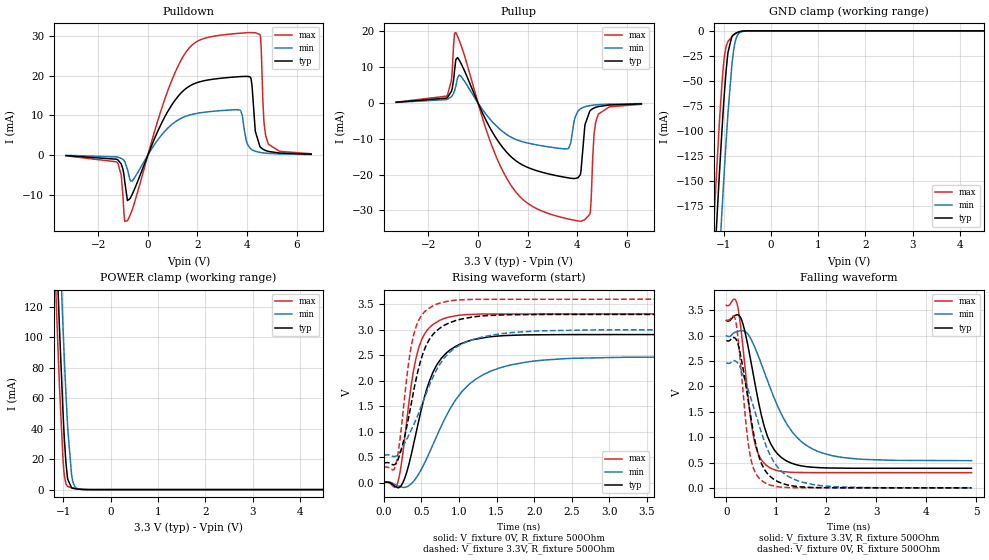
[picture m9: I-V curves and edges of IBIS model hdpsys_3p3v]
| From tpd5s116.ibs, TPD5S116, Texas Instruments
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[Model]   hdpsys_3p3v
Model_type   3-state
Polarity   Non-Inverting
Vmeas = 1.65
Vref = 3.3
Cref = 15pF
Rref = 500
|   typ   min   max
|   (nom PVT)   (slow PVT)   (fast PVT)
C_comp   1.1241p   1.0342p   1.3025p
|C_comp (High state)   1.1241p   1.0342p   1.3025p
|C_comp (Low state)   1.0197p   0.970p   1.0858p
| Where nom  PVT is Nominal Process, 3.3V, 27C
|   Fast PVT is Strong Process,  3.6V, -40C
|   Slow PVT is Weak Process,   3.0V, 125C
[Voltage Range]   3.3   3   3.6
[Temperature Range]   27   125   -40
[Pullup Reference]   3.3   3   3.6
[Pulldown Reference]   -0   -0   -0
[Power Clamp Reference]   3.3   3   3.6
[GND Clamp Reference]   -0   -0   -0
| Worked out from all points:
|   slope of the pulldown table from 0 to 0.495 V, typ, clamps not added: 68 ohm
|   slope of the pullup table from 0 to 0.495 V, typ, clamps not added: 69.7 ohm
|   GND clamp passes 1 mA (typ) near -0.67 V on its own axis
|   POWER clamp passes 1 mA (typ) near -0.81 V on its own axis
|   falling waveform, V_fixture 3.3V, R_fixture 500Ohm: 20-80 % time 394ps typ, 706ps min, 239ps max; typ from 3.3 V to 0.386 V
|   rising waveform, V_fixture 0V, R_fixture 500Ohm: 20-80 % time 342ps typ, 596ps min, 205ps max; typ from 0 V to 2.9 V
|   rising waveform, V_fixture 3.3V, R_fixture 500Ohm: 20-80 % time 285ps typ, 480ps min, 181ps max; typ from 0.386 V to 3.3 V
|   falling waveform, V_fixture 0V, R_fixture 500Ohm: 20-80 % time 325ps typ, 540ps min, 208ps max; typ from 2.91 V to 0 V
[Pulldown]
|   Voltage   I(typ)   I(min)   I(max)
-3.3V     -127.7uA   -60.24uA   -174.8uA
-1.261V   -1.034mA   -454.9uA   -1.695mA
-825mV    -11.44mA   -3.562mA   -16.52mA
-627mV    -9.783mA   -6.424mA   -13.66mA
1.492V    16.52mA    9.679mA    25.47mA
3.719V    19.73mA    11.3mA     30.64mA
4.125V    19.64mA    1.723mA    30.8mA
4.333V    5.994mA    958.9uA    30.76mA
4.531V    2.076mA    665.1uA    30.05mA
4.679V    1.346mA    539uA      8.703mA
4.858V    938uA      438.2uA    2.819mA
6.59V     231.5uA    153.5uA    329.1uA
[GND Clamp]
|   Voltage   I(typ)   I(min)   I(max)
-3.3V     -2.279A    -2.354A    -2.233A
-1.211V   -250.7mA   -335.6mA   -197.1mA
-1.102V   -155.4mA   -239.1mA   -103.5mA
-1.082V   -138.9mA   -222mA     -87.85mA
-1.033V   -99.21mA   -180.2mA   -52.35mA
-993.3mV  -70.07mA   -147.9mA   -30.38mA
-943.8mV  -39.09mA   -109.6mA   -15.28mA
-904.2mV  -21.17mA   -81.3mA    -10.57mA
-805.2mV  -4.668mA   -26.32mA   -5.052mA
-706.2mV  -1.575mA   -4.538mA   -1.734mA
-409.2mV  -5.798uA   -24.6uA    -1.856uA
6.59V     0A         0A         0A
[Pullup]
|   Voltage   I(typ)   I(min)   I(max)
-3.3V     179.2uA    152uA      210.7uA
-1.261V   1.394mA    952.3uA    1.976mA
-1.073V   3.233mA    1.738mA    6.287mA
-894.3mV  12.11mA    4.731mA    19.64mA
1.333V    -15.02mA   -9.557mA   -23.02mA
3.61V     -20.88mA   -12.8mA    -32.33mA
4.155V    -18.95mA   -1.528mA   -33.04mA
4.313V    -6.129mA   -1.045mA   -32.57mA
4.521V    -2.186mA   -732.1uA   -30.73mA
4.679V    -1.417mA   -594uA     -9.022mA
4.848V    -1.023mA   -494.1uA   -3.234mA
6.59V     -256.8uA   -177.9uA   -369.9uA
[POWER Clamp]
|   Voltage   I(typ)   I(min)   I(max)
-3.3V     2.245A     2.294A     2.215A
-1.191V   199.8mA    260.7mA    159.9mA
-1.142V   156.7mA    217.5mA    116.9mA
-1.082V   107.3mA    167.2mA    68.58mA
-1.003V   48.93mA    104.4mA    18.23mA
-973.5mV  31.29mA    82.8mA     8.212mA
-943.8mV  17.54mA    62.77mA    3.75mA
-904.2mV  6.605mA    39.45mA    2.019mA
-825mV    1.189mA    9.849mA    1.236mA
-805.2mV  935.2uA    6.339mA    1.111mA
-656.7mV  256.6uA    314.4uA    366uA
6.59V     0A         0A         0A
[Ramp]
R_load = 500
|   typ   min   max
dV/dt_r   1.74315/3.4176e-10   1.47905/5.96469e-10   1.98662/2.05392e-10
dV/dt_f   1.74853/3.94369e-10   1.47839/7.06289e-10   1.98031/2.39383e-10
[Falling Waveform]
V_fixture = 3.3V
V_fixture_min = 3V
V_fixture_max = 3.6V
R_fixture = 500Ohm
C_fixture = 0F
|   Time   V(typ)   V(min)   V(max)
0s        3.3V       3V         3.6V
215.6ps   3.414V     3.081V     3.627V
334.4ps   3.223V     3.097V     2.752V
460.3ps   2.655V     2.989V     1.571V
539.1ps   2.237V     2.837V     1.025V
657.2ps   1.626V     2.554V     626.7mV
805.8ps   1.065V     2.16V      439.2mV
1.222ns   522.9mV    1.238V     313.2mV
1.822ns   400.6mV    722.3mV    299.9mV
4.9ns     385.8mV    536mV      299.5mV
[Rising Waveform]
V_fixture = 0V
V_fixture_min = 0V
V_fixture_max = 0V
R_fixture = 500Ohm
C_fixture = 0F
|   Time   V(typ)   V(min)   V(max)
0s        5.238nV    193.4nV    1.486nV
161.8ps   -85.32mV   -49.23mV   -79.76mV
249.3ps   -9.314mV   -92.25mV   550.9mV
367.9ps   576.3mV    -17.03mV   1.959V
460.3ps   1.192V     163.3mV    2.631V
605.5ps   1.993V     589.7mV    3.04V
745.4ps   2.399V     1.052V     3.186V
1.132ns   2.781V     1.926V     3.298V
1.722ns   2.891V     2.319V     3.308V
4.9ns     2.905V     2.465V     3.311V
[Rising Waveform]
V_fixture = 3.3V
V_fixture_min = 3V
V_fixture_max = 3.6V
R_fixture = 500Ohm
C_fixture = 0F
|   Time   V(typ)   V(min)   V(max)
0s        385.5mV    535.3mV    299.4mV
149.8ps   359.2mV    511.3mV    307.7mV
249.3ps   746mV      700.5mV    1.309V
323.4ps   1.241V     910.1mV    2.293V
395ps     1.791V     1.131V     2.894V
525.9ps   2.563V     1.608V     3.327V
657.2ps   2.914V     2.083V     3.473V
951.2ps   3.177V     2.647V     3.578V
1.522ns   3.286V     2.913V     3.596V
4.9ns     3.3V       3V         3.6V
[Falling Waveform]
|Gnd
V_fixture = 0V
V_fixture_min = 0V
V_fixture_max = 0V
R_fixture = 500Ohm
C_fixture = 0F
|   Time   V(typ)   V(min)   V(max)
0s        2.905V     2.466V     3.311V
186.9ps   2.939V     2.498V     3.292V
269.4ps   2.691V     2.392V     2.603V
395ps     1.989V     2.054V     1.243V
460.3ps   1.577V     1.862V     723.7mV
605.5ps   783.5mV    1.396V     257.6mV
745.4ps   394.9mV    960.8mV    114.9mV
1.041ns   117.8mV    387.4mV    20.3mV
1.522ns   17.63mV    110.3mV    2.611mV
4.9ns     191.2uV    353.5uV    41.28uV
